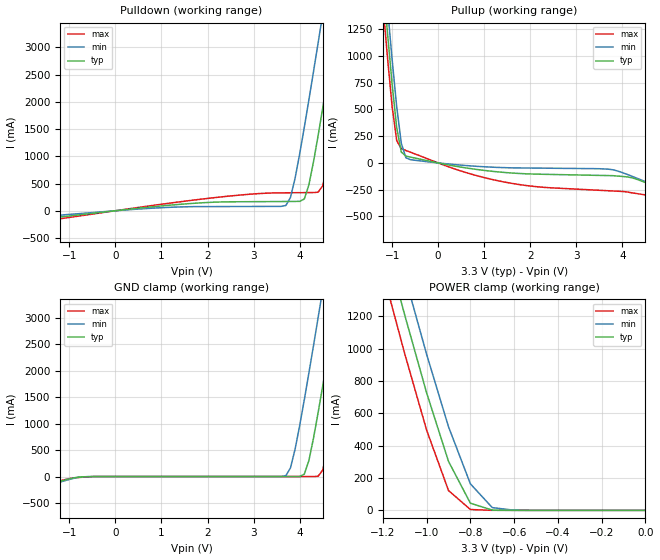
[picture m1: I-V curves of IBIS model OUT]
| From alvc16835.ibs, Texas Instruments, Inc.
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|   Model ALVC16835_OUT
[Model]   OUT
Model_type   3-state
Polarity   Non-Inverting
Enable   Active-High
|Variable   typ   min   max
C_comp   7.0pF   NA   NA
[Voltage range]   3.3   3.0   3.6
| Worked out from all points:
|   slope of the pulldown table from 0 to 0.495 V, typ, clamps not added: 10.8 ohm
|   slope of the pullup table from 0 to 0.495 V, typ, clamps not added: 12.6 ohm
|   GND clamp passes 1 mA (typ) near -0.52 V on its own axis
|   POWER clamp passes 1 mA (typ) near -0.66 V on its own axis
[Pullup]   | Note: Vtable = Vcc - Voutput
|   Voltage   I(typ)   I(min)   I(max)
-3.3V     13.15A     13.37A     12.95A
-1.2V     1.719A     1.96A      1.485A
-1.1V     1.216A     1.455A     987mA
-1V       740.3mA    970.5mA    530.9mA
-900mV    329.9mA    526.9mA    208.8mA
-800mV    101.6mA    183.9mA    133.9mA
-700mV    64.09mA    48.12mA    116.3mA
500mV     -39.59mA   -20.85mA   -76.07mA
1.4V      -87.63mA   -43.6mA    -175.5mA
3.8V      -119.5mA   -64.53mA   -262.5mA
4.7V      -218.3mA   -210.2mA   -320.6mA
6.6V      -566.3mA   -553mA     -685.1mA
[Pulldown]
|   Voltage   I(typ)   I(min)   I(max)
-3.3V     -427.6mA   -433.7mA   -424.2mA
-1.1V     -105.6mA   -74.03mA   -134.8mA
3.7V      169.7mA    96.85mA    329.3mA
3.8V      170.2mA    244.1mA    330.1mA
4V        172.7mA    1.045A     331.7mA
4.1V      215.7mA    1.531A     332.6mA
4.2V      474.7mA    2.038A     333.4mA
4.4V      1.38A      3.081A     340.2mA
4.5V      1.885A     3.612A     458.3mA
4.8V      3.465A     5.225A     1.81A
5.1V      5.084A     6.856A     3.396A
6.6V      13.34A     15.12A     11.64A
[POWER_Clamp]   | Note: Vtable = Vcc - Voutput
|   Voltage   I(typ)   I(min)   I(max)
-3.3V     13.15A     13.37A     12.95A
-1.2V     1.712A     1.957A     1.472A
-1.1V     1.207A     1.45A      967.4mA
-1V       726mA      964.2mA    495.9mA
-900mV    302.7mA    516.7mA    122.4mA
-800mV    44.2mA     164mA      5.222mA
-700mV    1.634mA    16.95mA    93.3uA
-600mV    43.98uA    914.4uA    883.8nA
0V        990pA      903.2pA    1.08nA
[GND_Clamp]
|   Voltage   I(typ)   I(min)   I(max)
-3.3V     -652mA     -663.5mA   -641mA
-800mV    -11.3mA    -15.06mA   -17.41mA
3.7V      34.64nA    16.95mA    1.13nA
3.9V      44uA       516.7mA    1.233nA
4.1V      44.2mA     1.45A      13.94nA
4.2V      302.7mA    1.957A     883.8nA
4.4V      1.207A     3A         5.222mA
4.5V      1.712A     3.53A      122.4mA
4.8V      3.29A      5.143A     1.472A
5.1V      4.908A     6.773A     3.055A
5.2V      5.451A     7.319A     3.594A
6.6V      13.15A     15.03A     11.28A
[Ramp]
| variable   typ   min   max
dV/dt_r   1.5677E+00/2.2126E-10  1.1516E+00/3.3528E-10  1.9139E+00/1.6698E-10
dV/dt_f   1.6333E+00/1.6391E-10  1.3640E+00/3.9882E-10  1.8664E+00/1.3165E-10
